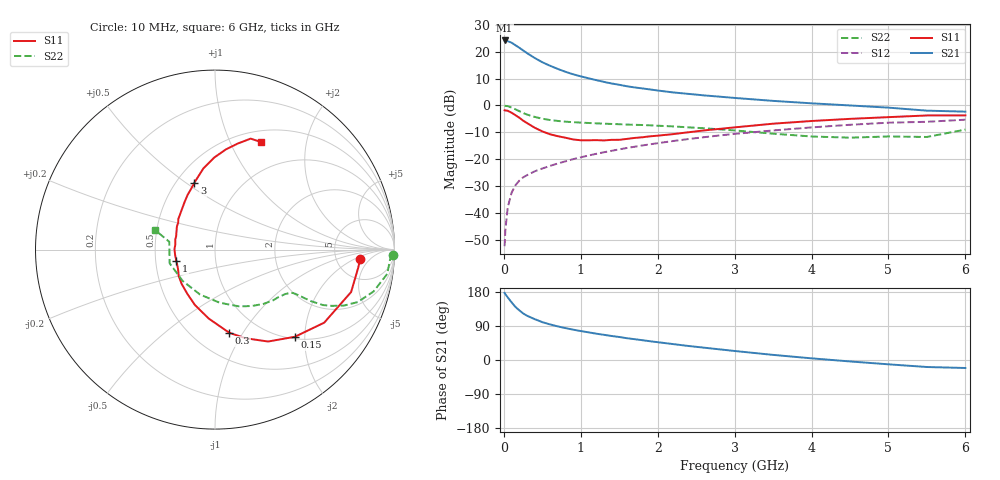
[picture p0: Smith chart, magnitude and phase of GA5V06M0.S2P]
! Infineon Technologies  Discrete & RF Semiconductors
! BF775
! Si NPN RF Bipolar Junction Transistor in SOT23
! VCE = 5 V  IC = 6 mA
! Common Emitter S-Parameters:  May  1996
# GHz  S  MA  R  50
!  f  S11  S21  S12  S22
! GHz  MAG  ANG  MAG  ANG  MAG  ANG  MAG  ANG
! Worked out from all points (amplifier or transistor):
!   36 points, 10 MHz to 6 GHz, reference 50 ohm
!   highest |S21| = 24.2 dB at 10 MHz (marker M1)
!   |S21| within 3 dB of that: start of sweep to 215.2 MHz
!   unconditionally stable (mu >= 1): 759.7 MHz to 3.162 GHz
!   at 250 MHz: K = 0.53, MSG = 23.6 dB, |S12| = -26.8 dB
!   at 1.4 GHz: K = 1.11, MAG = 10.5 dB, |S12| = -16.9 dB
!   at 6 GHz: K = 0.93, MSG = 1.5 dB, |S12| = -5.3 dB
!   S11 on the Smith chart (normalised r, x): 10 MHz: 8.74, -2.67; 150 MHz: 1.04, -1.79; 300 MHz: 0.73, -0.87; 1 GHz: 0.64, -0.09; 3 GHz: 0.61, +0.54; 6 GHz: 0.63, +1.32
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0.01  0.8106 -3.7  16.15 177.0  0.0024 88.9  0.9919 -1.6
0.02  0.8042 -7.2  16.02 173.6  0.0048 90.5  0.9768 -3.2
0.05  0.7944 -17.3  15.65 165.4  0.0125 81.8  0.9694 -8.0
0.1  0.732 -33.8  14.7 152.3  0.0236 74.3  0.9136 -14.8
0.15  0.6587 -47.5  13.2 140.3  0.0325 67.7  0.847 -20.2
0.2  0.5914 -60.0  11.84 131.2  0.0397 63.6  0.7827 -23.5
0.25  0.5216 -71.1  10.56 123.1  0.0457 61.4  0.7229 -25.7
0.3  0.47 -80.3  9.405 116.9  0.0502 59.9  0.6759 -27.2
0.4  0.3853 -95.3  7.647 107.9  0.0592 58.4  0.6106 -28.2
0.5  0.3281 -110.0  6.356 99.9  0.0669 58.6  0.5649 -28.5
0.6  0.2904 -122.1  5.469 93.9  0.0749 59.1  0.5342 -28.6
0.7  0.2674 -133.7  4.779 88.7  0.0828 59.5  0.5138 -28.8
0.8  0.2504 -143.9  4.22 84.2  0.0909 59.8  0.4981 -29.1
1  0.2244 -163.4  3.468 76.4  0.1081 60.4  0.4789 -30.4
1.1  0.2242 -172.1  3.193 73.0  0.1166 60.5  0.4706 -31.4
1.6  0.2378 154.3  2.269 57.5  0.1612 59.2  0.4394 -37.5
2.2  0.2918 129.0  1.743 42.0  0.2172 55.3  0.4064 -48.0
3  0.3898 107.2  1.376 23.8  0.2947 47.6  0.3421 -67.4
3.5  0.4565 98.2  1.213 13.5  0.3417 41.9  0.2975 -84.8
4.5  0.5615 83.8  0.997 -3.8  0.4357 29.3  0.2509 -135.9
5.5  0.6494 72.2  0.798 -18.5  0.4949 14.2  0.2584 170.3
6  0.6518 66.7  0.765 -21.1  0.5422 10.1  0.3548 161.7
